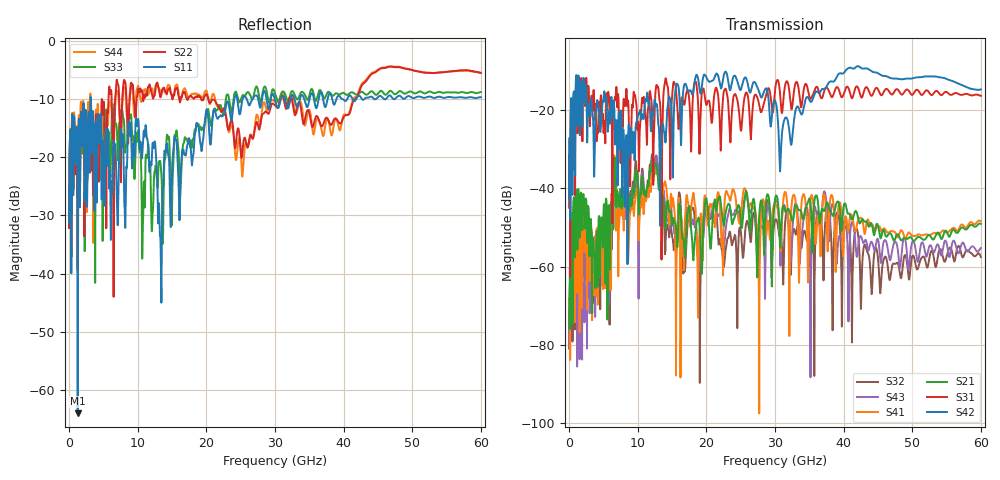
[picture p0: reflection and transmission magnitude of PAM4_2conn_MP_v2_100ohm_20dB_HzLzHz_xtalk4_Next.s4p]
! Info: Touchstone file created by Circ.  Input file=FAB50GbE_2conn_Midplane_Examax_Topo2_v2_100ohm_20dB_HzLzHz.circ
# Hz S RI R 50
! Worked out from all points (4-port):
!   6000 points, 10 MHz to 60 GHz, reference 50 ohm
!   strongest paths, dB at 10 MHz, 15.01 GHz, 30.01 GHz, 45.01 GHz, 60 GHz:
!     S42: -42.5, -25.2, -17.5, -10.5, -14.7
!     S31: -44.9, -16.5, -14.9, -14.6, -16.3
!     S21: -75.6, -49.5, -42.7, -49.5, -49.1
!     S41: -68.0, -44.7, -44.0, -49.6, -48.3
!     S43: -71.1, -48.3, -43.5, -53.0, -55.2
!     S32: -74.9, -52.2, -48.2, -57.9, -57.5
!   lowest |S11| = -63.9 dB at 1.26 GHz (marker M1), VSWR 1.00, Z = 50 - j0.0576 ohm
!   |S11| at or under -10 dB: start of sweep to 3.127 GHz; 3.184 GHz to 24.08 GHz (20.9 GHz wide, 153 % of centre); 29.97 GHz to 30.86 GHz (895.9 MHz wide, 2.95 % of centre)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
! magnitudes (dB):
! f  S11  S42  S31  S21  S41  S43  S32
! 10 MHz  -31.2  -42.5  -44.9  -75.6  -68.0  -71.1  -74.9
! 1.26 GHz  -63.9  -15.9  -20.4  -44.8  -48.2  -53.5  -50.7
! 12.67 GHz  -19.9  -18.8  -14.0  -33.7  -35.3  -32.4  -31.7
! 18.99 GHz  -16.2  -14.4  -31.0  -48.8  -51.8  -59.9  -68.4
! 21.17 GHz  -11.8  -11.7  -15.9  -43.3  -48.8  -43.5  -43.9
! 30.8 GHz  -10.3  -33.6  -17.0  -54.8  -55.4  -59.8  -52.0
! 60 GHz  -9.7  -14.7  -16.3  -49.1  -48.3  -55.2  -57.5
